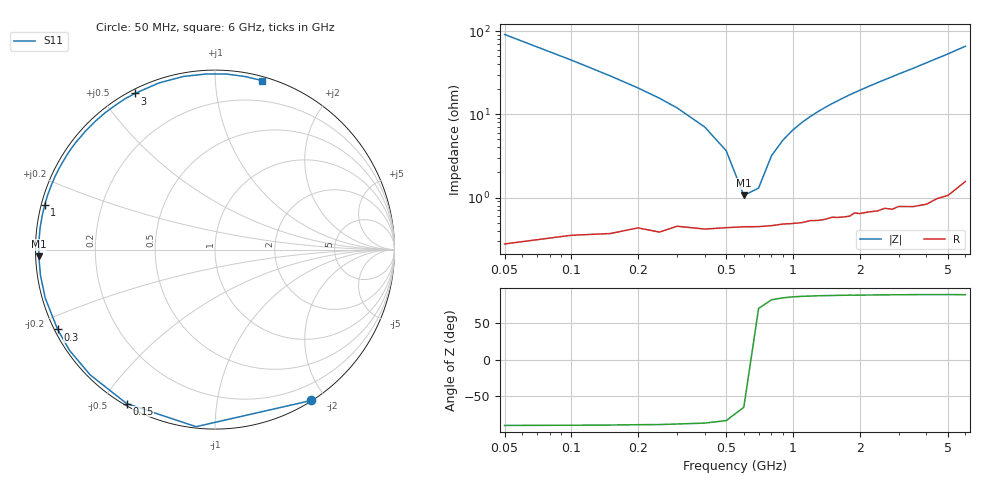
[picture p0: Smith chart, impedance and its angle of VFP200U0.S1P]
! Infineon Technologies  Discrete & RF Semiconductors
! BBY 58-03
! Si Tuning Diode in SOD323
! VR = 0.2 V
! S-Parameters:  June  1999
# GHz  S  MA  R  50
!  f  S11
! GHz  MAG  ANG
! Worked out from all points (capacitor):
!   34 points, 50 MHz to 6 GHz, reference 50 ohm
!   read as one part to ground: C = 34.6 pF near 50 MHz
!   lowest |Z| = 1.06 ohm at 600 MHz (marker M1)
!   series resonance near 644 MHz, so ESL is about 1.8 nH
!   S11 on the Smith chart (normalised r, x): 50 MHz: 0.01, -1.83; 150 MHz: 0.01, -0.58; 300 MHz: 0.01, -0.24; 1 GHz: 0.01, +0.13; 3 GHz: 0.02, +0.61; 6 GHz: 0.03, +1.32
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0.05  0.9974 -57.4
0.1  0.9922 -96.1
0.15  0.989 -119.8
0.2  0.9854 -134.9
0.25  0.9861 -145.3
0.3  0.983 -153.1
0.4  0.9838 -164.0
0.5  0.9829 -171.7
0.6  0.9824 -177.8
0.7  0.9823 177.2
0.8  0.9819 172.8
1  0.981 165.2
1.1  0.9807 161.8
1.3  0.9799 155.6
1.5  0.9786 149.9
1.6  0.979 147.3
1.8  0.9788 142.2
2  0.978 137.5
2.2  0.9776 133.0
2.4  0.9778 128.8
2.8  0.9784 120.9
3  0.9775 117.1
3.5  0.9797 108.6
4  0.9806 100.4
4.5  0.9796 93.0
5  0.9803 86.4
5.5  0.9788 80.0
6  0.9774 74.4
